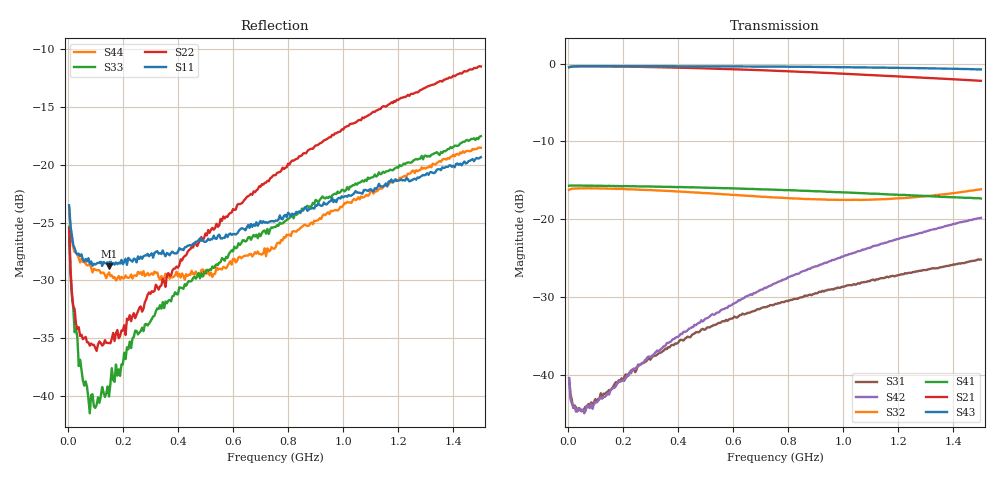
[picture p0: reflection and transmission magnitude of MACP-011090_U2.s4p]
!Agilent Technologies,E5071C,MY46110647,A.11.31
!Date: Tue Jan 18 13:58:20 2022 DD
!Data & Calibration Information:
!MACP-011090 soldered onto PT-0003645 with F connectors, Port1 (pin1) Port2 (pin6) Port3 (pin4) Port4 (pin3)
!Freq	S11:SOLT4(ON)	S12:SOLT4(ON)	S13:SOLT4(ON)	S14:SOLT4(ON)
!	S21:SOLT4(ON)	S22:SOLT4(ON)	S23:SOLT4(ON)	S24:SOLT4(ON)
!	S31:SOLT4(ON)	S32:SOLT4(ON)	S33:SOLT4(ON)	S34:SOLT4(ON)
!	S41:SOLT4(ON)	S42:SOLT4(ON)	S43:SOLT4(ON)	S44:SOLT4(ON)
!PortZ  Port1:75+j0  Port2:75+j0  Port3:75+j0  Port4:75+j0
!Above PortZ is port z conversion or system Z0 setting when saving the data.
!When reading, reference impedance value at option line is always used.
# Hz S MA R 75
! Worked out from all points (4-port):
!   300 points, 5 MHz to 1.5 GHz, reference 75 ohm
!   strongest paths, dB at 5 MHz, 380 MHz, 755 MHz, 1.13 GHz, 1.5 GHz:
!     S43: -0.5, -0.4, -0.4, -0.5, -0.8
!     S21: -0.5, -0.5, -0.9, -1.5, -2.2
!     S41: -15.7, -15.9, -16.2, -16.7, -17.3
!     S32: -16.2, -16.4, -17.2, -17.5, -16.2
!     S42: -40.4, -35.5, -28.2, -23.3, -19.8
!     S31: -40.5, -36.2, -30.9, -27.7, -25.2
!   lowest |S11| = -28.8 dB at 150 MHz (marker M1), VSWR 1.08, Z = 70.5 + j2.86 ohm
!   |S11| at or under -10 dB: start of sweep to end of sweep
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5000000  0.06681 145.2  0.948 2.2  0.01021 153.8  0.1653 179.8
         0.9479 2.2  0.05329 124.0  0.1527 3.7  0.009538 144.7
         0.009457 152.9  0.1544 4.2  0.05393 122.8  0.9471 2.5
         0.164 -179.8  0.009524 152.6  0.9465 2.3  0.06512 140.4
3e7  0.04172 156.1  0.9596 -0.5  0.005674 151.7  0.1644 177.4
     0.9598 -0.5  0.02055 128.7  0.1575 0.7  0.005997 172.2
     0.006165 150.7  0.1575 0.7  0.01963 139.8  0.9586 -0.2
     0.1643 177.4  0.005786 171.3  0.9597 -0.1  0.04168 162.4
8e7  0.03735 156.7  0.9606 -2.9  0.006636 137.4  0.1641 172.9
     0.9607 -2.9  0.01653 125.6  0.1578 -0.8  0.006811 -172.4
     0.006366 138.2  0.1578 -0.8  0.008439 176.6  0.9613 -2.0
     0.1642 173.0  0.006115 -171.8  0.9608 -2.0  0.03711 173.2
1.5e8  0.03636 146.2  0.9581 -5.7  0.007824 119.6  0.1633 166.8
       0.9585 -5.7  0.01698 107.9  0.157 -2.1  0.008219 -164.7
       0.007987 120.3  0.157 -2.1  0.00997 -152.2  0.9609 -4.1
       0.1637 166.9  0.007452 -164.2  0.9607 -4.1  0.03427 179.8
2.45e8  0.03903 132.1  0.954 -9.5  0.01108 98.3  0.1627 158.7
        0.9537 -9.5  0.02173 76.4  0.1551 -3.5  0.01128 -163.2
        0.01039 103.5  0.155 -3.4  0.01921 -123.2  0.9607 -6.8
        0.1626 158.8  0.01091 -164.5  0.9608 -6.8  0.03324 -168.5
6.2e8  0.05147 70.5  0.9176 -23.5  0.02438 62.1  0.1574 127.0
       0.9171 -23.6  0.0677 9.3  0.1425 -5.8  0.02978 162.6
       0.02373 63.5  0.1426 -5.6  0.04583 -98.5  0.9575 -17.5
       0.1573 127.2  0.03017 162.6  0.958 -17.5  0.03979 -137.3
1.5e9  0.1078 -28.1  0.7753 -52.9  0.05709 6.3  0.1357 55.5
       0.7744 -52.8  0.2656 -67.2  0.1548 9.2  0.1017 78.7
       0.05505 6.9  0.1554 9.5  0.1328 -98.6  0.9145 -44.7
       0.1358 56.6  0.102 80.3  0.9171 -44.7  0.1184 -130.9
